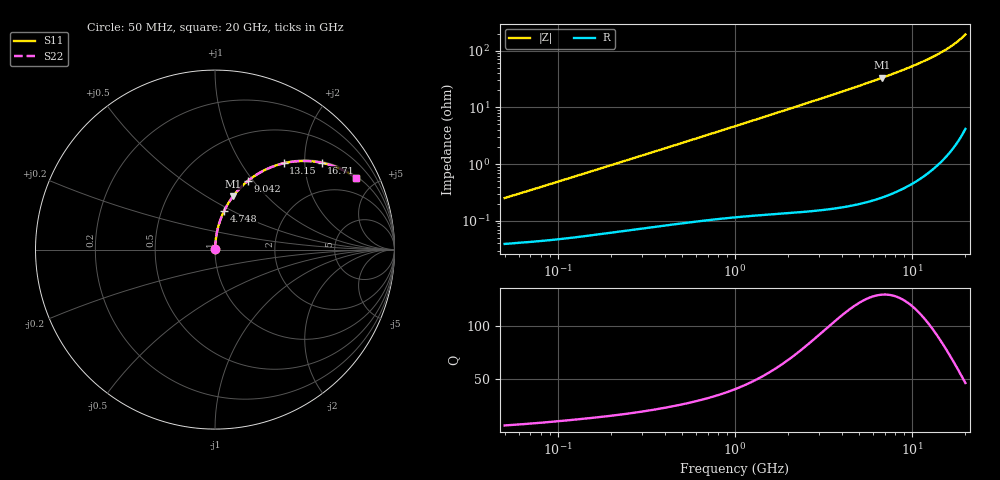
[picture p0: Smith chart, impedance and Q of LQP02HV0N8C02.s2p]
!Murata Part Number: LQP02HV0N8C02
!These Parameters are Measured in Series Mode Connection
!  o--[Z]--o
!Port1  Port2
!  o-------o
!Freq. Start=50[MHz] Stop=20[GHz], 401[Steps]
# Hz S RI R 50
!Freq.(Hz) S11(Real) S11(Imag) S21(Real) S21(Imag) S12(Real) S12(Imag) S22(Real) S22(Imag)
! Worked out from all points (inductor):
!   401 points, 50 MHz to 20 GHz, reference 50 ohm
!   read as one part in series: L = 786 pH near 51.52 MHz
!   highest Q = 129 at 6.802 GHz (marker M1), where L = 782 pH
!   S11 on the Smith chart (normalised r, x): 50 MHz: 1.00, +0.00; 4.748 GHz: 1.00, +0.45; 9.042 GHz: 1.01, +0.94; 13.15 GHz: 1.02, +1.57; 16.71 GHz: 1.04, +2.43; 20 GHz: 1.08, +3.87
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5e7  0.000398 0.00249  0.9996 -0.00249  0.9996 -0.00249  0.000398 0.00249
6.166548e7  0.000421 0.00305  0.9996 -0.00305  0.9996 -0.00305  0.000421 0.00305
1.364002e8  0.000572 0.00659  0.9994 -0.00659  0.9994 -0.00659  0.000572 0.00659
3.721004e8  0.00111 0.0176  0.9989 -0.0176  0.9989 -0.0176  0.00111 0.0176
1e9  0.00331 0.0464  0.9967 -0.0464  0.9967 -0.0464  0.00331 0.0464
1.714689e9  0.00761 0.079  0.9924 -0.079  0.9924 -0.079  0.00761 0.079
2.728004e9  0.0174 0.125  0.9826 -0.125  0.9826 -0.125  0.0174 0.125
3.626126e9  0.0298 0.1652  0.9702 -0.1652  0.9702 -0.1652  0.0298 0.1652
4.748272e9  0.0502 0.2143  0.9498 -0.2143  0.9498 -0.2143  0.0502 0.2143
5.769027e9  0.0738 0.2575  0.9262 -0.2575  0.9262 -0.2575  0.0738 0.2575
6.802353e9  0.1025 0.2994  0.8975 -0.2994  0.8975 -0.2994  0.1025 0.2994
7.442007e9  0.1226 0.3242  0.8774 -0.3242  0.8774 -0.3242  0.1226 0.3242
9.041845e9  0.1814 0.3813  0.8186 -0.3813  0.8186 -0.3813  0.1814 0.3813
1.004137e10  0.2239 0.4127  0.7761 -0.4127  0.7761 -0.4127  0.2239 0.4127
1.098561e10  0.268 0.4385  0.732 -0.4385  0.732 -0.4385  0.268 0.4385
1.201863e10  0.3204 0.4619  0.6796 -0.4619  0.6796 -0.4619  0.3204 0.4619
1.314879e10  0.3821 0.4807  0.6179 -0.4807  0.6179 -0.4807  0.3821 0.4807
1.504638e10  0.4933 0.4939  0.5067 -0.4939  0.5067 -0.4939  0.4933 0.4939
1.670968e10  0.5946 0.4838  0.4054 -0.4838  0.4054 -0.4838  0.5946 0.4838
1.800918e10  0.6728 0.4609  0.3272 -0.4609  0.3272 -0.4609  0.6728 0.4609
1.940974e10  0.7525 0.4217  0.2475 -0.4217  0.2475 -0.4217  0.7525 0.4217
2e10  0.7839 0.4009  0.2161 -0.4009  0.2161 -0.4009  0.7839 0.4009
